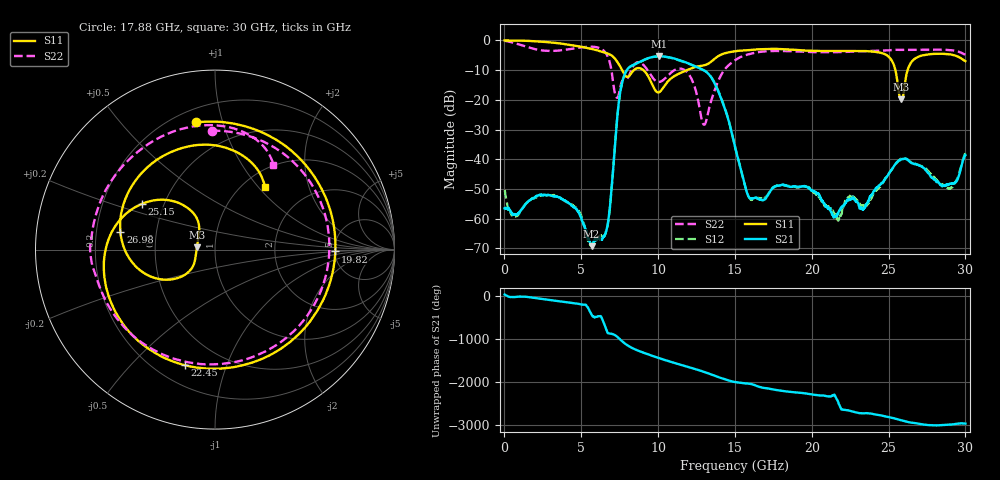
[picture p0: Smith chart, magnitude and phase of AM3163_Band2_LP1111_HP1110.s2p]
!Agilent Technologies,E8364B,MY43040894,A.07.50.67
!Agilent E8364B: A.07.50.67
!Date: Thursday, August 20, 2020 12:08:20
!Correction: S11(Full 2 Port(1,2))
!S21(Full 2 Port(1,2))
!S12(Full 2 Port(1,2))
!S22(Full 2 Port(1,2))
!S2P File: Measurements: S11, S21, S12, S22:
# Hz S  dB  R 50
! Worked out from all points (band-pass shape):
!   3201 points, 10 MHz to 30 GHz, reference 50 ohm
!   highest |S21| = -5.38 dB at 10.07 GHz (marker M1); lowest = -69.2 dB at 5.671 GHz (marker M2)
!   |S21| within 3 dB of the highest: 8.332 GHz to 12.25 GHz (3.918 GHz wide, 38.1 % of centre)
!   lowest |S11| = -19.8 dB at 25.83 GHz (marker M3), VSWR 1.23, Z = 40.8 + j1.11 ohm
!   |S11| at or under -10 dB: 7.658 GHz to 8.421 GHz (762.7 MHz wide, 9.49 % of centre); 9.039 GHz to 11.88 GHz (2.838 GHz wide, 27.1 % of centre); 25.44 GHz to 26.24 GHz (794.4 MHz wide, 3.07 % of centre)
!   |S22| runs from -28.4 to -0.1 dB; largest |S21 - S12| = 0.0079
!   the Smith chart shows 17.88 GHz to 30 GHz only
!   S11 on the Smith chart (normalised r, x): 17.88 GHz: 0.28, +0.82; 19.82 GHz: 5.06, -0.19; 22.45 GHz: 0.31, -0.73; 25.15 GHz: 0.38, +0.25; 26.98 GHz: 0.30, +0.08; 30 GHz: 1.24, +1.09
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1e7  -0.03 -2.6  -56.55 43.3  -50.36 32.4  -0.14 -6.5
1.978094e9  -0.29 -71.4  -52.75 -36.2  -53.00 -36.3  -2.93 -171.2
3.411991e9  -0.91 -124.1  -52.59 -107.9  -52.44 -107.7  -3.49 84.1
5.014581e9  -2.16 171.7  -60.23 170.8  -59.22 177.8  -2.34 -20.1
5.670612e9  -2.88 140.4  -69.24 -66.3  -69.01 17.2  -2.12 -63.0
6.701519e9  -4.41 76.2  -62.52 -119.7  -62.61 -137.3  -5.23 -154.2
7.788656e9  -11.27 -12.7  -11.90 -4.7  -11.97 -4.5  -13.15 -87.4
8.772703e9  -9.33 -80.0  -7.34 165.0  -7.39 165.5  -7.38 -130.5
1.000979e10  -17.52 -161.8  -5.39 7.0  -5.40 7.2  -13.99 -161.1
1.006602e10  -17.44 -161.2  -5.38 0.4  -5.39 0.6  -14.00 -159.7
1.158427e10  -10.66 74.7  -6.99 -167.0  -7.09 -166.2  -9.64 148.8
1.300879e10  -8.38 -36.2  -10.15 38.3  -10.14 39.6  -28.38 -95.7
1.5005e10  -3.65 -128.7  -35.85 163.9  -35.73 163.5  -6.70 -112.3
1.788217e10  -2.90 98.3  -48.83 -32.5  -48.93 -34.6  -3.57 91.7
1.982214e10  -3.47 -0.9  -49.62 -115.6  -49.49 -114.7  -3.92 -1.2
2.000958e10  -3.51 -9.7  -50.53 -125.5  -50.48 -122.5  -3.94 -9.4
2.244627e10  -3.53 -104.5  -53.75 -143.1  -52.73 -150.9  -3.84 -97.8
2.500479e10  -5.48 157.6  -44.94 65.8  -44.87 66.9  -3.35 -167.6
2.515474e10  -6.36 148.1  -43.84 54.6  -43.86 55.7  -3.26 -171.4
2.582952e10  -19.85 172.4  -40.04 -9.3  -39.72 -8.5  -3.20 170.1
2.698226e10  -5.41 169.5  -42.12 -89.6  -42.02 -88.3  -3.18 140.6
3e10  -6.98 51.5  -38.62 -86.0  -37.90 -82.1  -4.81 55.5
